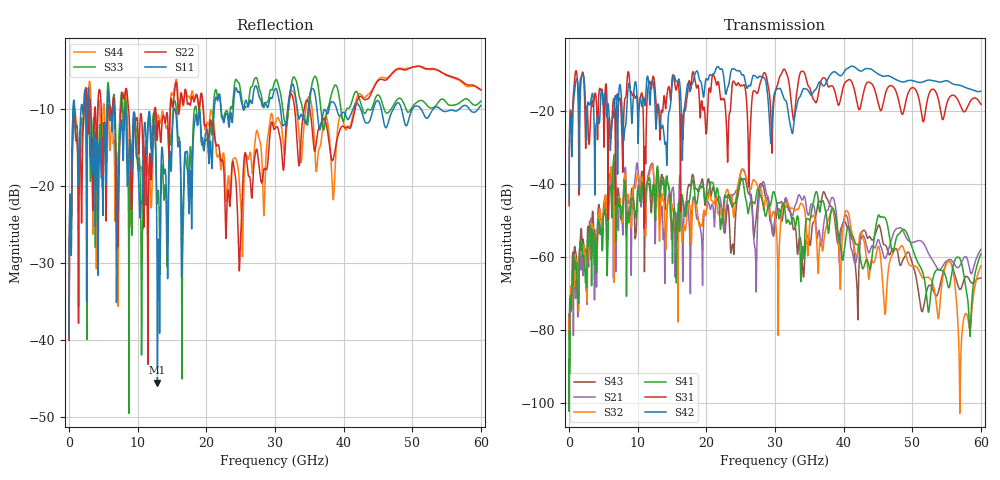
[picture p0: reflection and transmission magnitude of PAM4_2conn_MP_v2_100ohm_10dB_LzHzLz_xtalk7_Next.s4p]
! Info: Touchstone file created by Circ.  Input file=FAB50GbE_2conn_Midplane_Examax_Topo2_v2_100ohm_10dB_LzHzLz.circ
# Hz S RI R 50
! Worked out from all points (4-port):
!   6000 points, 10 MHz to 60 GHz, reference 50 ohm
!   strongest paths, dB at 10 MHz, 15.01 GHz, 30.01 GHz, 45.01 GHz, 60 GHz:
!     S42: -44.7, -13.0, -14.7, -9.9, -14.7
!     S31: -46.0, -11.2, -15.2, -17.7, -18.3
!     S41: -88.0, -55.1, -43.1, -48.8, -59.2
!     S32: -82.5, -45.7, -49.0, -57.2, -62.5
!     S21: -75.6, -41.5, -48.8, -55.3, -57.9
!     S43: -77.3, -52.8, -51.1, -51.5, -65.7
!   lowest |S11| = -45.6 dB at 12.88 GHz (marker M1), VSWR 1.01, Z = 50.3 + j0.428 ohm
!   |S11| at or under -10 dB: 8.2 GHz to 15.3 GHz (7.102 GHz wide, 60.4 % of centre); 15.43 GHz to 21.15 GHz (5.72 GHz wide, 31.3 % of centre); 54.1 GHz to 56.86 GHz (2.756 GHz wide, 4.97 % of centre)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
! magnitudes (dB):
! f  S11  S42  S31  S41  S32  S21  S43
! 10 MHz  -39.6  -44.7  -46.0  -88.0  -82.5  -75.6  -77.3
! 960 MHz  -12.2  -12.2  -9.2  -63.0  -65.1  -71.2  -58.9
! 6.1 GHz  -10.9  -27.4  -27.3  -41.7  -35.8  -37.8  -39.5
! 12.88 GHz  -45.6  -19.1  -20.3  -35.2  -41.2  -37.1  -36.2
! 40.49 GHz  -11.2  -8.5  -11.8  -52.5  -47.4  -48.9  -51.8
! 57.07 GHz  -9.8  -13.1  -18.8  -61.0  -87.5  -61.9  -68.8
! 60 GHz  -9.5  -14.7  -18.3  -59.2  -62.5  -57.9  -65.7
